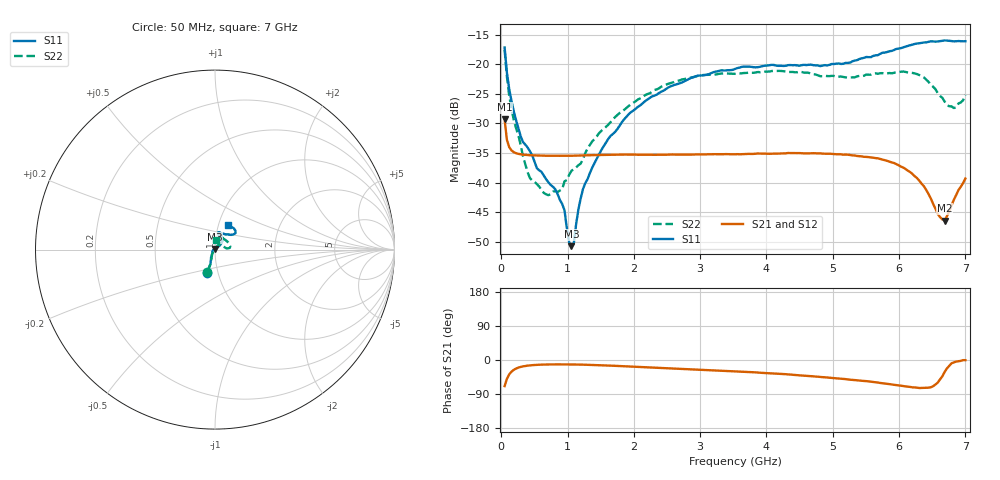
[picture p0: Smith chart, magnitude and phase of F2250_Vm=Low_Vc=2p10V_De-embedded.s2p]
! Integrated Device Technology
! Corporate Headquarters
! 6024 Silver Creek Valley Road
! San Jose, CA 95138  USA
! Phone:  1-408-284-8200
! Toll Free:  1-800-223-1366
! Webpage:  http://www.idt.com/
! Timing and RF Division
! 515 Groton Road, Suite 102
! Westford, MA 01886-6024
! Device:  F2250
! Description: Voltage Variable RF Attenuator
! Frequency:  50.0 -  6000.00 MHz
! Package:  3x3 mm Thin QFN Plastic Package: 16 pin
! Ports:  2 RF, 3 DC
!  Pin  1  = GND
!  Pin  2  = NC
!  Pin  3  = RF1  = Port 1
!  Pin  4  = NC
!  Pin  5  = GND
!  Pin  6  = GND
!  Pin  7  = GND
!  Pin  8  = GND
!  Pin  9  = NC
!  Pin 10  = RF2  = Port 2
!  Pin 11  = NC
!  Pin 12  = GND
!  Pin 13  = GND
!  Pin 14  = VCNTRL
!  Pin 15  = VDD
!  Pin 16  = VMODE
! Vcntrl:  2.100 Volts
! Vmode:  +0.000 Volts
! Vdd:  +3.30  Volts
! Current:  1.180 mA
! Data:  The device was measured on a the F2250 evaluation board which has
!  individual transmission lines to the RF pins.  Data was collected
!  using a calibrated network analyzer.  The evaluation board was
!  de-embedded using a TRL calibration technique.
!  The reference plane is the edge of the package pin.
! Misc:  SN 10
!  Action Tracker AT0258
! Date Measured:  2014-11-26
! Date:  2015-10-15  MJV
! Note:
!  Integrated Device Technology supplies this data as a sample of measured
!  data at the package pin for this product.  Your particular data for this
!  product may vary.
!  Data was taken at 25 degrees C.
!  Integrated Device Technology reserves the right to change this data at anytime.
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# GHz S dB R 50
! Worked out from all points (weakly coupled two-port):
!   201 points, 50 MHz to 7 GHz, reference 50 ohm
!   highest |S21| = -29.34 dB at 50 MHz (marker M1); lowest = -46.4 dB at 6.687 GHz (marker M2)
!   lowest |S11| = -50.7 dB at 1.058 GHz (marker M3), VSWR 1.01, Z = 49.8 + j0.243 ohm
!   |S11| at or under -10 dB: start of sweep to end of sweep
!   |S22| runs from -42.1 to -17.6 dB; largest |S21 - S12| = 5.4e-05
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0.05  -17.18 -108.6  -29.34 -69.0  -29.34 -69.0  -17.55 -109.7
0.08475  -21.44 -107.4  -32.78 -49.6  -32.78 -49.6  -22.16 -107.0
0.189  -28.00 -119.7  -34.87 -25.8  -34.86 -25.9  -29.45 -119.3
0.29325  -32.21 -127.8  -35.23 -18.2  -35.23 -18.2  -33.72 -126.2
0.43225  -34.71 -144.6  -35.38 -14.1  -35.38 -14.1  -39.24 -159.2
0.71025  -39.96 -168.5  -35.47 -11.8  -35.46 -11.8  -42.13 145.7
0.91875  -43.61 158.1  -35.47 -11.6  -35.48 -11.6  -41.12 111.8
0.9535  -44.68 169.4  -35.48 -11.6  -35.48 -11.6  -39.79 111.9
1.023  -50.06 144.1  -35.47 -11.7  -35.47 -11.7  -38.70 93.1
1.05775  -50.74 122.8  -35.46 -11.7  -35.46 -11.8  -38.02 88.4
1.0925  -50.39 89.8  -35.45 -11.8  -35.45 -11.8  -37.74 83.3
1.162  -44.60 56.6  -35.43 -12.0  -35.43 -12.0  -37.07 72.4
1.2315  -41.11 44.0  -35.41 -12.3  -35.40 -12.3  -36.09 64.3
1.6485  -32.11 41.9  -35.33 -14.9  -35.32 -14.9  -29.80 53.9
2.37825  -24.87 47.3  -35.29 -20.6  -35.28 -20.6  -24.08 51.4
3.525  -20.80 72.5  -35.22 -30.0  -35.22 -30.1  -21.63 72.0
4.7065  -20.17 72.4  -35.03 -43.1  -35.04 -43.1  -21.69 70.7
5.85325  -17.82 40.4  -36.45 -63.7  -36.45 -63.8  -21.49 20.1
6.33975  -16.40 41.0  -40.19 -73.8  -40.20 -73.9  -22.00 6.0
6.68725  -15.99 48.8  -46.41 -31.3  -46.38 -30.9  -26.33 26.1
6.861  -16.12 55.1  -42.10 -4.2  -42.05 -4.2  -27.28 58.3
7  -16.12 63.3  -39.32 -0.4  -39.28 -0.5  -25.19 85.2
